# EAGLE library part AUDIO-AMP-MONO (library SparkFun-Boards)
SparkFun Mono Audio Amp Breakout- TPA2005D1 This tiny audio amplifier is based on the Texas Instruments TPA2005D1. Its efficient class-D operation means low heat and long battery life. It can drive an 8-Ohm speaker at up to 1.4 Watts SparkFun Products: Mono Audio Amp Breakout
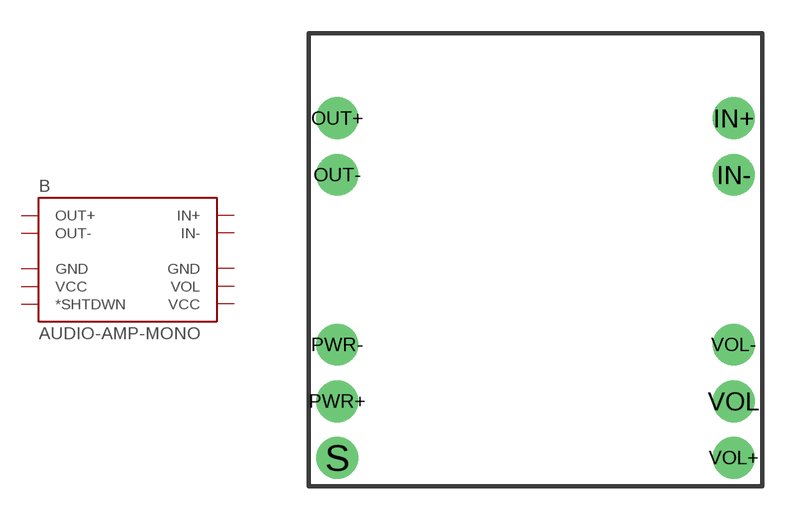
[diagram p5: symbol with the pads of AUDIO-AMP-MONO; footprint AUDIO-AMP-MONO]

Designator prefix B

## AUDIO-AMP-MONODIP  [AUDIO-AMP-MONO]
IN+  IN+
IN-  IN-
OUT+  OUT+
OUT-  OUT-
PWR+  VCC
PWR-  GND
S  *SHTDWN
VOL  VOL
VOL+  VCC
VOL-  GND

## Footprint AUDIO-AMP-MONO (pad centres in mm)
drill 1.016 pad 1.88: IN+ 8.89,6.35; IN- 8.89,3.81; OUT+ -8.89,6.35; OUT- -8.89,3.81; PWR+ -8.89,-6.35; PWR- -8.89,-3.81; S -8.89,-8.89; VOL 8.89,-6.35; VOL+ 8.89,-8.89; VOL- 8.89,-3.81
